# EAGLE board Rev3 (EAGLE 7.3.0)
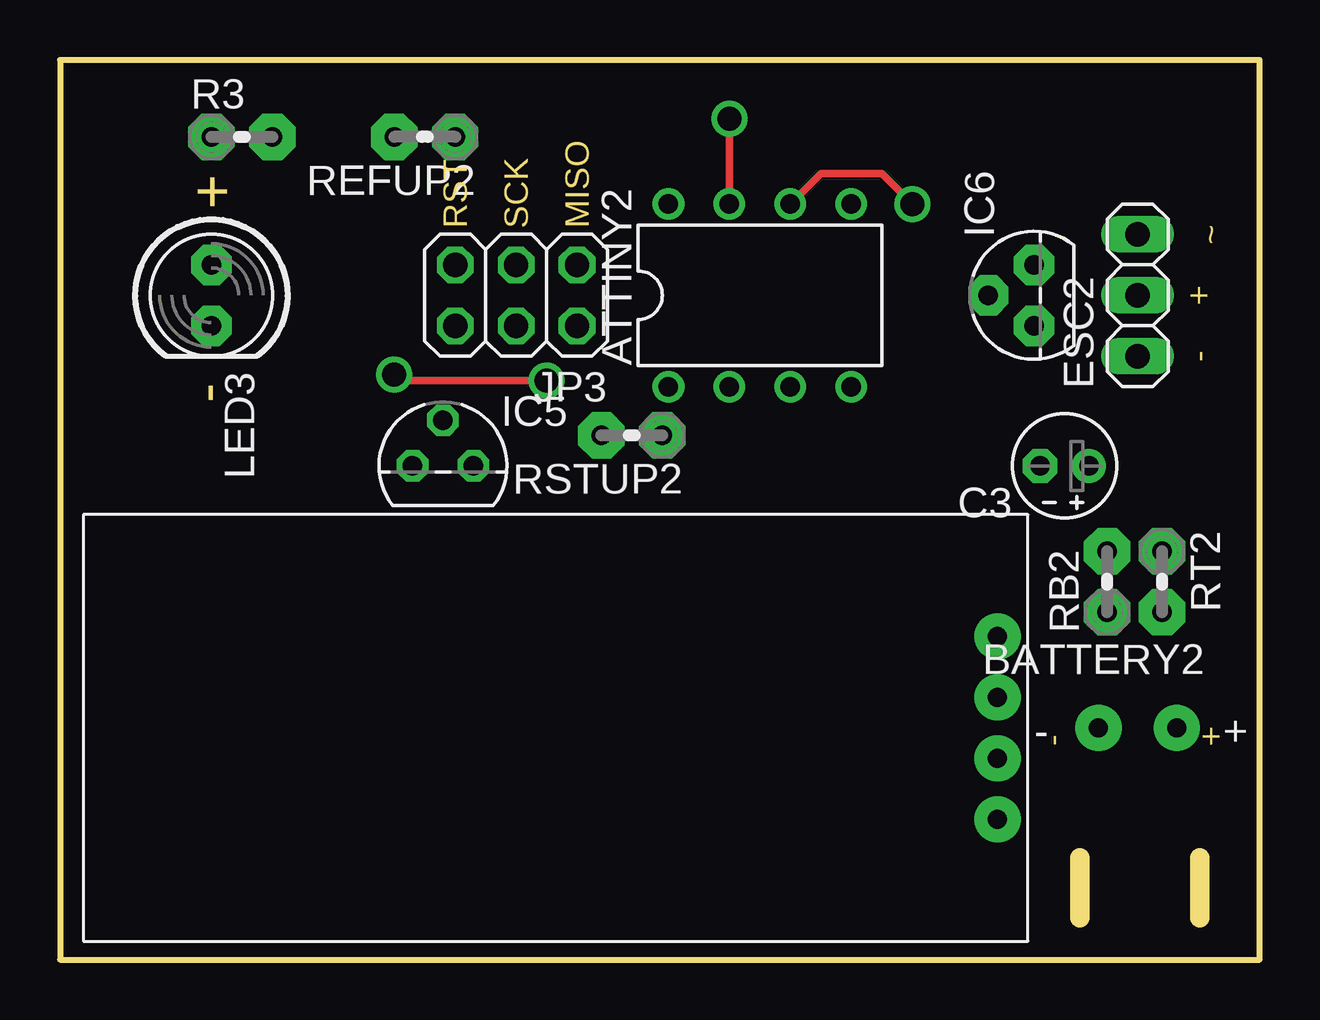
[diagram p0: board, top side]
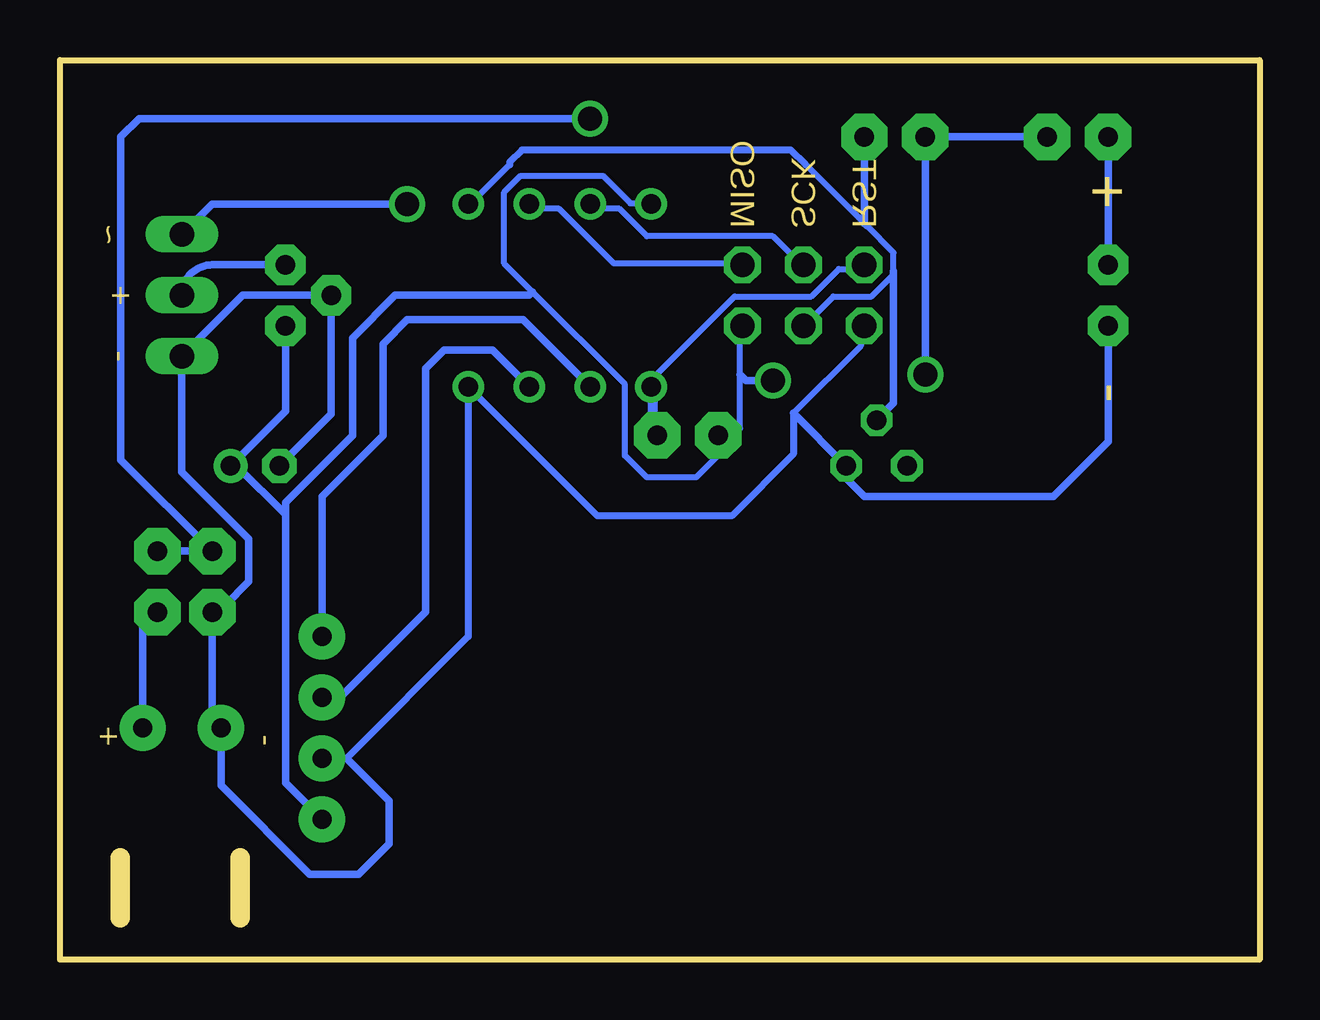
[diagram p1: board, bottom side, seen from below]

Size 50 x 37.5 mm. Coordinates in mm from the lower left corner, seen from the top.
Outline: 0,0 50,0 50,37.5 0,37.5 0,0
Copper layers (1*16): Top 0.035mm / dielectric 1.5mm / Bottom 0.035mm
Design rules "default": minimum track width 10mil, minimum drill 24mil, track to track 8mil, track to pad 8mil, pad to pad 8mil, via to via 8mil, smd to smd 8mil, copper to edge 40mil, drill to drill 8mil, minimum pad ring 10mil, minimum via ring 8mil, stop-mask expansion 4mil, vias tented up to drill 0mil, thermal gap 10mil
Milling: 2 lines

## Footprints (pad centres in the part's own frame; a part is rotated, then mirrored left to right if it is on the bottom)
DIL08 = drill 0.813 pad 1.27: 1 -3.81,-3.81; 2 -1.27,-3.81; 3 1.27,-3.81; 4 3.81,-3.81; 5 3.81,3.81; 6 1.27,3.81; 7 -1.27,3.81; 8 -3.81,3.81
JST-PH-2-THM = drill 0.8 pad 1.93: 1 1.635,0; 2 -1.635,0
E2-4 = drill 0.813 pad 1.422: + -1.016,0 | drill 0.813 pad 1.422 octagon: - 1.016,0
1X03 = drill 1.016 long: 1 -2.54,0; 2 0,0; 3 2.54,0
BT = drill 0.8 pad 1.93: GND -1.27,0; RX 3.81,0; TX 1.27,0; VCC -3.81,0
TO92 = drill 0.813 octagon: 1 -1.27,0; 2 0,1.905; 3 1.27,0
TO92' = drill 0.813 pad 1.676 octagon: 1 -1.27,0; 2 0,1.905; 3 1.27,0
2X03 = drill 1.016 octagon: 1 -2.54,-1.27; 2 -2.54,1.27; 3 0,-1.27; 4 0,1.27; 5 2.54,-1.27; 6 2.54,1.27
LED5MM = drill 0.813 pad 1.676 octagon: A -1.27,0; K 1.27,0
0204V = drill 0.813 pad 1.93 octagon: 1 -1.27,0; 2 1.27,0

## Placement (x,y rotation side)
ATTINY2  ATTINY45DIP8  [DIL08]  29.17,27.69 0 top
BATTERY2  [JST-PH-2-THM]  44.92,9.66 180 top
C3  0.1uf  [E2-4]  41.87,20.58 180 top
ESC2  [1X03]  44.92,27.69 90 top
HC-02  HC-O6  [BT]  39.08,9.66 90 top
IC5  LM336LP  [TO92]  15.96,20.58 0 top
IC6  78L05Z  [TO92']  40.6,27.69 90 top
JP3  [2X03]  19.01,27.69 180 top
LED3  [LED5MM]  6.31,27.69 270 top
R3  270  [0204V]  7.58,34.29 0 top
RB2  20000  [0204V]  43.65,15.75 90 top
REFUP2  2200  [0204V]  15.2,34.29 180 top
RSTUP2  10000  [0204V]  23.84,21.85 180 top
RT2  220000  [0204V]  45.94,15.75 270 top

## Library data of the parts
ATTINY2 HC-02 IC5 = VLADLIBRARY
BATTERY2 C3 IC6 LED3 R3 RB2 REFUP2 RSTUP2 RT2 = adafruit
ESC2 JP3 = pinhead

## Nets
CONTROL2: ATTINY2.6 ESC2.3 JP3.1
GND2: ATTINY2.4 BATTERY2.1 C3.- ESC2.1 HC-02.GND IC5.3 IC6.2 JP3.6 LED3.K RB2.1
N$9: ATTINY2.1 JP3.5 RSTUP2.1
N$10: ESC2.2 IC6.3
N$11: BATTERY2.2 RT2.2
N$12: LED3.A R3.1
RX2: ATTINY2.3 HC-02.TX
TX2: ATTINY2.2 HC-02.RX
VCC2: ATTINY2.8 C3.+ HC-02.VCC IC6.1 JP3.2 R3.2 REFUP2.2 RSTUP2.2
VOLTMETER2: ATTINY2.7 JP3.3 RB2.2 RT2.1
VREF2: ATTINY2.5 IC5.2 JP3.4 REFUP2.1

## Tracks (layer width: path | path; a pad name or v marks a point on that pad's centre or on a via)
CONTROL2  (via drill 1)
  Top 0.305: v35.52,31.5 34.25,32.77 31.71,32.77 ATTINY2.6
  Bottom 0.254: ATTINY2.6 30.34,31.3 29.2,31.3 26.91,29.01 21.65,29.01 JP3.1
  Bottom 0.305: ESC2.3 43.65,31.5 v35.52,31.5
GND2
  Bottom 0.254: 19.43,22.77 16.62,25.58 16.62,26.27 JP3.6
  Bottom 0.3: 19.43,22.77 19.43,21.07 22,18.5 27.6,18.5 ATTINY2.4 32.98,13.47 38.06,8.39
  Bottom 0.305: 19.43,22.77 IC5.3 17.23,20.07 16.47,19.31 8.6,19.31 6.31,21.59 LED3.K | C3.- 38.7,22.74 IC6.2 42.38,27.69 ESC2.1 44.92,20.32 42.13,17.53 42.13,15.75 43.14,14.74 43.4,14.74 RB2.1 43.65,9.93 BATTERY2.1 43.28,7.26 39.59,3.56 37.55,3.56 36.28,4.83 36.28,6.61 38.06,8.39 HC-02.GND
N$9
  Bottom 0.254: 25.31,23.75 ATTINY2.1 25.54,23.98 21.88,27.64 18.68,27.64 17.54,28.78 16.62,28.78 JP3.5
  Bottom 0.406: 25.31,23.75 25.31,21.85 RSTUP2.1
N$10
  Bottom 0.305: IC6.3 43.65,28.96 arc-90 ESC2.2
N$11
  Bottom 0.305: BATTERY2.2 46.55,13.86 RT2.2
N$12
  Bottom 0.305: LED3.A R3.1
RX2
  Bottom 0.305: HC-02.TX 38.32,10.93 34.76,14.48 34.76,24.64 34,25.4 31.97,25.4 ATTINY2.3
TX2
  Bottom 0.305: HC-02.RX 39.08,19.31 36.54,21.85 36.54,25.66 35.52,26.67 30.7,26.67 ATTINY2.2
VCC2  (via drill 1)
  Top 0.305: v13.93,24.39 14.19,24.13 v20.28,24.13
  Bottom 0.254: ATTINY2.8 25.54,31.52 26.23,31.52 27.37,32.67 30.8,32.67 31.48,31.98 31.48,29.01 30.3,27.83 26.45,23.98 26.45,21.01 25.54,20.09 23.48,20.09 22.57,21.01 RSTUP2.2 22.57,21.24 21.65,22.15 21.65,24.39 21.65,26.27 JP3.2
  Bottom 0.305: R3.2 REFUP2.2 v13.93,24.39 | v20.28,24.13 21.4,24.13 21.65,24.39 | IC6.1 40.6,22.86 C3.+ 42.63,20.58 40.6,18.55 | HC-02.VCC 40.6,7.37 40.6,18.55 | 40.6,18.55 40.6,19.05 37.81,21.85 37.81,25.91 36.03,27.69 30.44,27.69 30.3,27.83
VOLTMETER2  (via drill 1 pad 1.27)
  Top 0.305: v27.9,35.06 ATTINY2.7
  Bottom 0.254: ATTINY2.7 27.83,31.3 26.68,31.3 25.54,30.15 20.28,30.15 19.14,29.01 JP3.3
  Bottom 0.305: RT2.1 RB2.2 47.46,20.83 47.46,34.29 46.7,35.06 v27.9,35.06
VREF2
  Bottom 0.254: 31.25,33.13 32.85,31.52 ATTINY2.5 | 18.91,33.13 16.37,30.59 15.25,29.47 15.25,28.71 15.25,28.55 16.17,27.64 17.77,27.64 18.91,26.5 JP3.4
  Bottom 0.3: 18.91,33.13 19.54,33.75 30.75,33.75 31.25,33.24 31.25,33.13
  Bottom 0.305: IC5.2 15.25,23.19 15.25,28.71 | REFUP2.1 16.47,30.69 16.37,30.59

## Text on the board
Milling: + | RST | SCK | MISO | ~ | + | - | - | - | +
